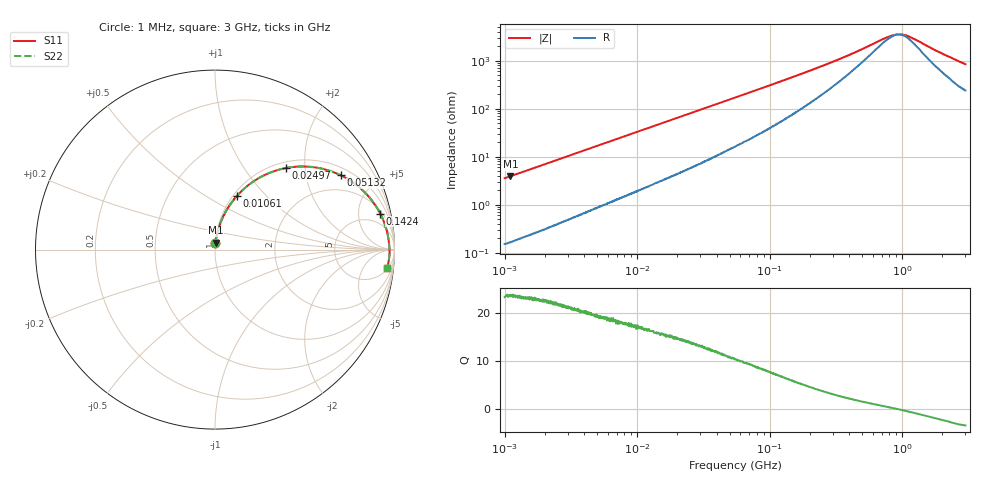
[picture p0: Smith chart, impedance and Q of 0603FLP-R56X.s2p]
!s-Parameter Generated by FASTRON Sdn. Bhd.
!FASTRON P/N : 0603FLP-R56X
!Keysight Technologies: E4991B_MY54100416_A.01.15
!Date: Tue Dec 02 12:51:50 2025
!Version  :Rev00  Tue Dec 02 12:51:50 2025
!Data & Calibration Information:
!Freq  S11  S21  S12  S22
!PortZ  Port1:50+j0  Port2:50+j0
!When reading reference impedance value at option line is always used.
! Remarks : This data is being provided solely for informational purposes.
# Hz S dB R 50
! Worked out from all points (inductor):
!   1601 points, 1 MHz to 3 GHz, reference 50 ohm
!   read as one part in series: L = 559 nH near 1.041 MHz
!   highest Q = 23.8 at 1.105 MHz (marker M1), where L = 561 nH
!   self-resonance near 935.3 MHz
!   S11 on the Smith chart (normalised r, x): 1 MHz: 1.00, +0.07; 10.61 MHz: 1.04, +0.70; 24.97 MHz: 1.12, +1.59; 51.32 MHz: 1.29, +3.18; 142.4 MHz: 2.40, +8.62; 3 GHz: 6, -16
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1000000  -29.00 85.5  -0.02 -2.0  -0.02 -2.0  -29.00 85.5
1105259  -28.20 85.4  -0.02 -2.2  -0.02 -2.2  -28.20 85.4
2118264  -22.80 83.3  -0.05 -4.2  -0.05 -4.2  -22.80 83.3
3804036  -17.90 79.9  -0.12 -7.3  -0.12 -7.3  -17.90 79.9
6696013  -13.30 74.5  -0.31 -12.4  -0.31 -12.4  -13.30 74.5
1.061086e7  -9.80 67.8  -0.65 -18.8  -0.65 -18.8  -9.80 67.8
1.447069e7  -7.62 61.9  -1.07 -24.5  -1.07 -24.5  -7.62 61.9
1.886552e7  -5.94 55.9  -1.62 -30.2  -1.62 -30.2  -5.94 55.9
2.49671e7  -4.40 48.9  -2.43 -37.0  -2.43 -37.0  -4.40 48.9
3.526298e7  -2.90 39.9  -3.84 -45.6  -3.84 -45.6  -2.90 39.9
5.132264e7  -1.78 30.5  -5.86 -54.2  -5.86 -54.2  -1.78 30.5
5.504702e7  -1.62 28.8  -6.30 -55.7  -6.30 -55.7  -1.62 28.8
8.636184e7  -0.90 19.7  -9.39 -63.6  -9.39 -63.6  -0.90 19.7
1.424433e8  -0.52 12.3  -13.30 -68.4  -13.30 -68.4  -0.52 12.3
2.083556e8  -0.38 8.3  -16.60 -69.1  -16.60 -69.1  -0.38 8.3
3.91407e8  -0.29 3.9  -22.50 -62.3  -22.50 -62.3  -0.29 3.9
7.925923e8  -0.25 0.7  -30.30 -22.0  -30.30 -22.0  -0.25 0.7
9.209708e8  -0.24 0.1  -31.20 -2.3  -31.20 -2.3  -0.24 0.1
1.002744e9  -0.24 -0.3  -31.20 10.6  -31.20 10.6  -0.24 -0.3
1.086329e9  -0.24 -0.6  -30.70 22.0  -30.70 22.0  -0.24 -0.6
1.86495e9  -0.26 -3.2  -24.10 60.3  -24.10 60.3  -0.26 -3.2
3e9  -0.34 -6.2  -18.90 67.3  -18.90 67.3  -0.34 -6.2
